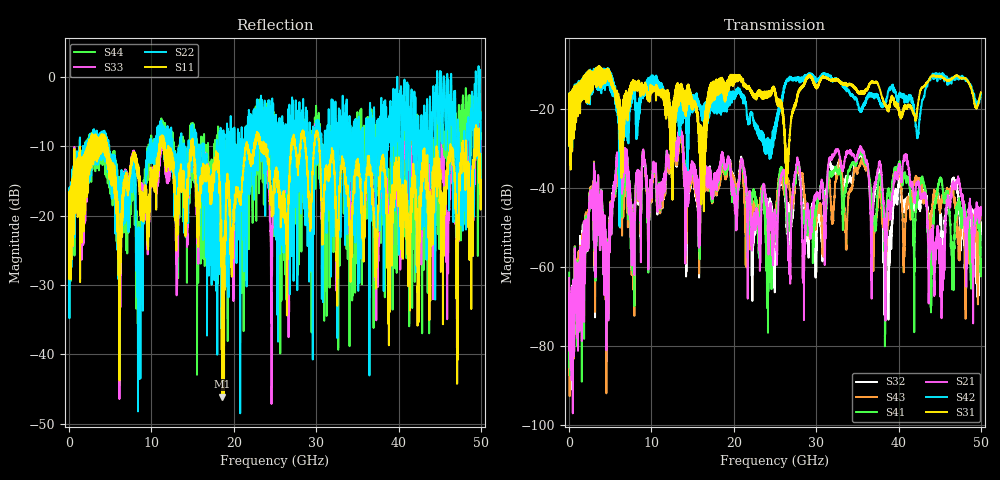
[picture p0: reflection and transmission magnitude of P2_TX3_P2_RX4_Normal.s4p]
!Keysight Technologies,N5225B,MY57041031,A.13.20.10
!Date: Friday, May 31, 2019 11:32:37
!Correction: S11(Full 4 Port(1,2,3,4))
!S12(Full 4 Port(1,2,3,4))
!S13(Full 4 Port(1,2,3,4))
!S14(Full 4 Port(1,2,3,4))
!S21(Full 4 Port(1,2,3,4))
!S22(Full 4 Port(1,2,3,4))
!S23(Full 4 Port(1,2,3,4))
!S24(Full 4 Port(1,2,3,4))
!S31(Full 4 Port(1,2,3,4))
!S32(Full 4 Port(1,2,3,4))
!S33(Full 4 Port(1,2,3,4))
!S34(Full 4 Port(1,2,3,4))
!S41(Full 4 Port(1,2,3,4))
!S42(Full 4 Port(1,2,3,4))
!S43(Full 4 Port(1,2,3,4))
!S44(Full 4 Port(1,2,3,4))
!S4P File: Measurements: <S11,S12,S13,S14>,
!<S21,S22,S23,S24>,
!<S31,S32,S33,S34>,
!<S41,S42,S43,S44>:
# Hz S  dB  R 50.0
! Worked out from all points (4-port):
!   5000 points, 10 MHz to 50 GHz, reference 50 ohm
!   strongest paths, dB at 10 MHz, 12.51 GHz, 25.01 GHz, 37.51 GHz, 50 GHz:
!     S31: -19.5, -42.1, -16.0, -13.6, -15.7
!     S42: -19.7, -27.8, -23.9, -16.9, -16.1
!     S21: -62.6, -28.9, -46.4, -35.2, -46.8
!     S41: -61.3, -29.2, -47.5, -39.2, -58.0
!     S43: -71.4, -30.1, -48.1, -43.1, -46.0
!     S32: -64.8, -29.8, -58.3, -35.5, -48.6
!   lowest |S11| = -46.1 dB at 18.62 GHz (marker M1), VSWR 1.01, Z = 49.7 - j0.379 ohm
!   |S11| at or under -10 dB: 4.63 GHz to 10.95 GHz (6.318 GHz wide, 81.1 % of centre); 15.13 GHz to 21.46 GHz (6.33 GHz wide, 34.6 % of centre); 30.38 GHz to 44.61 GHz (14.23 GHz wide, 37.9 % of centre)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
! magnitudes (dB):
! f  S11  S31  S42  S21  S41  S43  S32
! 10 MHz  -19.6  -19.5  -19.7  -62.6  -61.3  -71.4  -64.8
! 2.79 GHz  -11.7  -14.7  -15.9  -45.0  -44.1  -43.7  -44.4
! 4.58 GHz  -9.5  -10.0  -9.9  -62.6  -61.6  -66.4  -64.8
! 5.9 GHz  -18.5  -19.1  -20.1  -32.5  -34.0  -35.7  -34.0
! 18.62 GHz  -46.1  -12.3  -15.5  -32.4  -32.8  -34.3  -33.6
! 24.27 GHz  -13.4  -15.8  -27.6  -52.8  -51.8  -47.1  -44.9
! 50 GHz  -15.9  -15.7  -16.1  -46.8  -58.0  -46.0  -48.6
